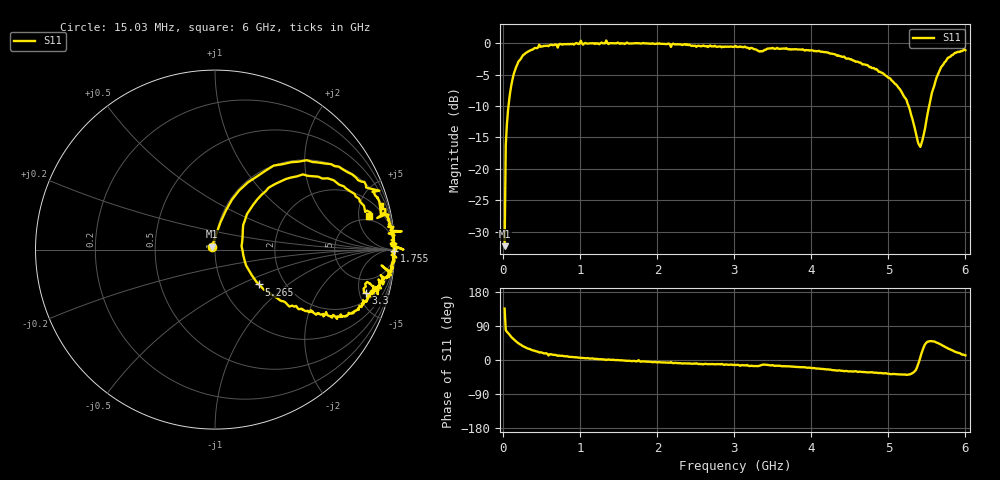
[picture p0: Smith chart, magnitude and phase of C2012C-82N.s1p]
!	Network	Analyzer	HP8753E.07.74:	Oct	30	2002	Serial	No.	JP38451487
!	Hewlett-Packard
!	7	Sep	2009	12:10:09
!	Frequency	S11
#	HZ	S	RI	R	50
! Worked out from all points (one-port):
!   400 points, 15.03 MHz to 6 GHz, reference 50 ohm
!   lowest |S11| = -32.3 dB at 15.03 MHz (marker M1), VSWR 1.05, Z = 48.3 + j1.63 ohm
!   |S11| at or under -10 dB: start of sweep to 65.59 MHz; 5.262 GHz to 5.53 GHz (268.1 MHz wide, 4.97 % of centre)
!   S11 on the Smith chart (normalised r, x): 15.03 MHz: 0.97, +0.03; 1.755 GHz: open; 3.3 GHz: 2.82, -5.76; 5.265 GHz: 1.48, -0.64; 6 GHz: 4.19, +6.79
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1.502992e7  -0.0173 0.0169
3.002985e7  0.0299 0.151
7.502962e7  0.135 0.33
1.350293e8  0.327 0.468
2.550287e8  0.647 0.476
4.650277e8  0.916 0.328
5.550272e8  0.905 0.292
5.850271e8  0.925 0.197
7.650262e8  0.954 0.19
1.005025e9  1.04 0.102
1.035025e9  0.968 0.0894
1.335023e9  1.05 6.1e-05
1.515022e9  0.987 -0.0126
1.755021e9  1 -0.00751
1.785021e9  0.989 -0.0787
2.265019e9  0.971 -0.139
3.015015e9  0.925 -0.216
3.300014e9  0.84 -0.241
3.375013e9  0.848 -0.18
3.765011e9  0.851 -0.264
4.515007e9  0.646 -0.372
5.025005e9  0.414 -0.317
5.265004e9  0.245 -0.194
5.415003e9  0.148 0.0196
5.535002e9  0.212 0.249
5.685002e9  0.49 0.419
5.865001e9  0.778 0.31
6e9  0.858 0.186
